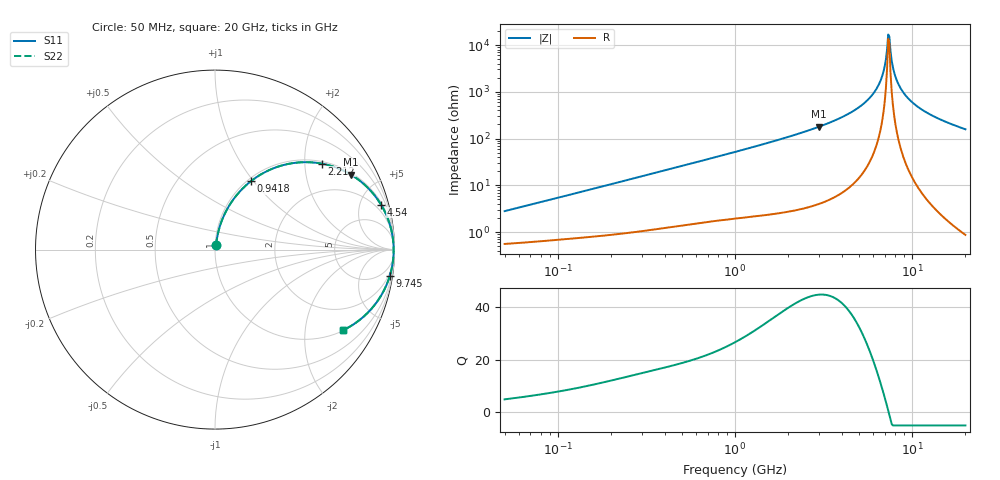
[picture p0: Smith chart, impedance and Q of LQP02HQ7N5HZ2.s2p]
!Murata Part Number: LQP02HQ7N5HZ2
!These Parameters are Measured in Series Mode Connection
!  o--[Z]--o
!Port1  Port2
!  o-------o
!Freq. Start=50[MHz] Stop=20[GHz], 401[Steps]
# Hz S RI R 50
!Freq.(Hz) S11(Real) S11(Imag) S21(Real) S21(Imag) S12(Real) S12(Imag) S22(Real) S22(Imag)
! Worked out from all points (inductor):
!   401 points, 50 MHz to 20 GHz, reference 50 ohm
!   read as one part in series: L = 8.7 nH near 51.52 MHz
!   highest Q = 44.7 at 2.985 GHz (marker M1), where L = 9.55 nH
!   self-resonance near 7.331 GHz
!   S11 on the Smith chart (normalised r, x): 50 MHz: 1.01, +0.06; 941.8 MHz: 1.04, +0.97; 2.212 GHz: 1.06, +2.44; 4.54 GHz: 1.20, +7.33; 9.745 GHz: 1, -13; 20 GHz: 1.02, -3.16
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5e7  0.0063 0.0272  0.9937 -0.0272  0.9937 -0.0272  0.0063 0.0272
1.364002e8  0.0127 0.0713  0.9873 -0.0713  0.9873 -0.0713  0.0127 0.0713
3.721004e8  0.0466 0.1827  0.9534 -0.1827  0.9534 -0.1827  0.0466 0.1827
9.418449e8  0.2006 0.3815  0.7994 -0.3815  0.7994 -0.3815  0.2006 0.3815
1e9  0.2196 0.3956  0.7804 -0.3956  0.7804 -0.3956  0.2196 0.3956
2.211938e9  0.5968 0.4787  0.4032 -0.4787  0.4032 -0.4787  0.5968 0.4787
2.728004e9  0.7116 0.4419  0.2884 -0.4419  0.2884 -0.4419  0.7116 0.4419
2.98453e9  0.7577 0.4175  0.2423 -0.4175  0.2423 -0.4175  0.7577 0.4175
4.539627e9  0.9249 0.2505  0.0751 -0.2505  0.0751 -0.2505  0.9249 0.2505
5.515528e9  0.9697 0.1537  0.0303 -0.1537  0.0303 -0.1537  0.9697 0.1537
6.311513e9  0.9876 0.0833  0.0124 -0.0833  0.0124 -0.0833  0.9876 0.0833
6.802353e9  0.993 0.0435  0.00696 -0.0435  0.00696 -0.0435  0.993 0.0435
7.009217e9  0.9943 0.0275  0.00571 -0.0275  0.00571 -0.0275  0.9943 0.0275
7.222371e9  0.995 0.0115  0.00499 -0.0115  0.00499 -0.0115  0.995 0.0115
7.442007e9  0.9952 -0.00458  0.00479 0.00458  0.00479 0.00458  0.9952 -0.00458
7.554318e9  0.9951 -0.0126  0.00488 0.0126  0.00488 0.0126  0.9951 -0.0126
7.901521e9  0.9941 -0.0366  0.00595 0.0366  0.00595 0.0366  0.9941 -0.0366
8.264682e9  0.9918 -0.0606  0.00819 0.0606  0.00819 0.0606  0.9918 -0.0606
8.907419e9  0.9854 -0.1004  0.0146 0.1004  0.0146 0.1004  0.9854 -0.1004
9.745021e9  0.9735 -0.1476  0.0265 0.1476  0.0265 0.1476  0.9735 -0.1476
1.314879e10  0.8991 -0.2955  0.1009 0.2955  0.1009 0.2955  0.8991 -0.2955
2e10  0.7129 -0.4496  0.2871 0.4496  0.2871 0.4496  0.7129 -0.4496
